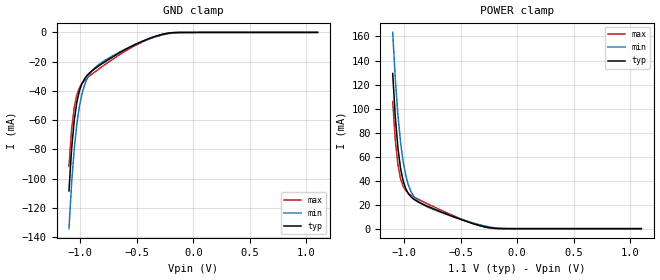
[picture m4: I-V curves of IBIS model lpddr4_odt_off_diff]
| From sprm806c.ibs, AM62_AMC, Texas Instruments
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|   Model lpddr4_odt_off_diff
[Model] lpddr4_odt_off_diff
Model_type Input
Polarity   Non-Inverting
Enable   Active-High
Vinl =  0.113V
Vinh =  0.253V
C_comp   2.469pF   2.415pF   2.634pF
[Model Spec]
Vinh   0.253V   0.247V   0.265V
Vinl   0.113V   0.107V   0.125V
[Temperature Range]   25.000   0.125k   -40.000
[Voltage Range]   1.100V   1.060V   1.170V
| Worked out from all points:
|   GND clamp passes 1 mA (typ) near -0.25 V on its own axis
|   POWER clamp passes 1 mA (typ) near -0.26 V on its own axis
[GND_clamp]
|Voltage   I(typ)   I(min)   I(max)
-1.1V     -108.4mA   -134.2mA   -91.64mA
-1.077V   -80.16mA   -103.8mA   -66.64mA
-1.054V   -60.67mA   -80.45mA   -51.43mA
-1.031V   -48.01mA   -63.14mA   -42.84mA
-1.008V   -40.05mA   -50.74mA   -37.98mA
-985mV    -35.04mA   -42.03mA   -35mA
-940mV    -29.42mA   -31.64mA   -31.25mA
-848mV    -23.51mA   -22.73mA   -25.72mA
-527mV    -8.751mA   -8.697mA   -9.53mA
-367mV    -3.504mA   -3.875mA   -3.689mA
-229mV    -630.6uA   -1.042mA   -565.6uA
1.1V      0A         0A         0A
[POWER_clamp]
|Voltage   I(typ)   I(min)   I(max)
-1.1V     129.2mA    163.4mA    105.9mA
-1.077V   92.86mA    124.8mA    73.42mA
-1.054V   67.3mA     94.72mA    53.18mA
-1.031V   50.48mA    72.24mA    41.68mA
-1.008V   39.92mA    56.02mA    35.38mA
-985mV    33.39mA    44.59mA    31.77mA
-963mV    29.32mA    36.69mA    29.55mA
-917mV    24.76mA    27.37mA    26.62mA
-871mV    22.09mA    22.56mA    24.32mA
-619mV    11.99mA    11.76mA    13.14mA
-229mV    602.8uA    1.183mA    400.8uA
1.1V      0A         0A         0A
